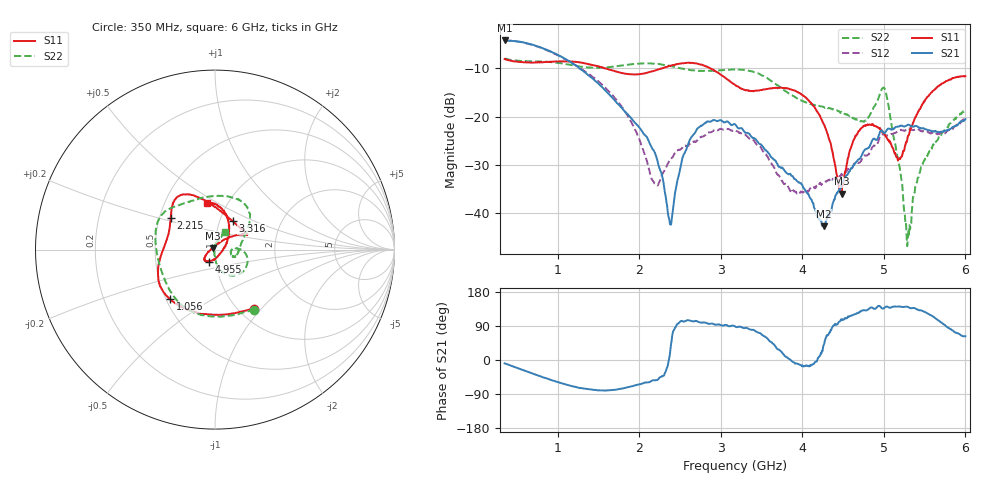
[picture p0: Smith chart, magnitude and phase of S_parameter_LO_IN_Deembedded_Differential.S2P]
!Agilent Technologies,E5071B,MY42403504,A.06.51
!Date: Mon Mar 10 15:44:32 2014
!Data & Calibration Information:
!Freq	S11:SOLT2(ON)	S21:SOLT2(ON)	S12:SOLT2(ON)	S22:SOLT2(ON)
# Hz S dB R 50
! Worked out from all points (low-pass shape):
!   801 points, 350 MHz to 6 GHz, reference 50 ohm
!   highest |S21| = -4.23 dB at 350 MHz (marker M1); lowest = -42.8 dB at 4.263 GHz (marker M2)
!   |S21| within 3 dB of the highest: start of sweep to 1.003 GHz
!   lowest |S11| = -36.0 dB at 4.482 GHz (marker M3), VSWR 1.03, Z = 48.7 + j0.937 ohm
!   |S11| at or under -10 dB: 1.579 GHz to 2.283 GHz (704.5 MHz wide, 36.5 % of centre); 2.871 GHz to end of sweep
!   |S22| runs from -46.8 to -8.0 dB; largest |S21 - S12| = 0.032
!   S11 on the Smith chart (normalised r, x): 350 MHz: 1.17, -0.91; 1.056 GHz: 0.53, -0.34; 2.215 GHz: 0.57, +0.22; 3.316 GHz: 1.15, +0.38; 4.955 GHz: 0.93, -0.13; 6 GHz: 0.81, +0.45
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3.5e8  -8.09 -56.4  -4.23 -8.8  -4.23 -8.4  -7.97 -56.8
1.05625e9  -8.57 -132.0  -7.69 -61.7  -7.82 -60.3  -9.01 -126.1
1.296375e9  -8.85 -150.0  -10.37 -74.3  -10.22 -72.2  -9.67 -146.9
1.826062e9  -11.10 173.2  -18.98 -73.7  -18.98 -83.5  -9.33 166.1
2.2145e9  -10.36 144.4  -28.61 -53.2  -34.12 -6.9  -9.10 144.2
2.235688e9  -10.22 143.1  -30.03 -50.2  -33.98 7.1  -9.10 143.0
2.384e9  -9.46 135.6  -42.37 29.3  -28.77 47.8  -9.55 135.1
2.52525e9  -8.95 129.2  -28.97 103.2  -26.51 63.7  -10.06 126.5
2.645312e9  -8.89 123.1  -24.15 102.3  -25.35 74.4  -10.43 117.5
3.175e9  -13.46 80.0  -21.58 88.5  -22.87 97.0  -10.24 66.5
3.31625e9  -14.52 58.7  -23.38 85.0  -23.96 94.1  -10.43 55.8
3.853e9  -14.34 26.4  -31.84 0.5  -35.47 35.5  -15.44 22.0
4.121375e9  -17.48 35.4  -37.65 -11.8  -34.87 40.0  -17.41 -1.3
4.262625e9  -21.58 45.1  -42.76 39.6  -33.75 53.5  -18.04 -12.5
4.481562e9  -35.98 142.8  -33.96 105.2  -31.85 80.7  -19.04 -21.5
4.679312e9  -23.36 -144.3  -29.05 124.1  -29.61 107.9  -20.63 -16.2
4.95475e9  -22.40 -116.8  -23.10 141.1  -24.11 140.6  -15.23 -7.9
5.060688e9  -24.89 -95.6  -22.47 138.9  -23.78 137.0  -18.08 -74.1
5.194875e9  -28.63 -33.1  -22.01 141.2  -22.86 140.9  -30.56 -97.6
5.300812e9  -23.89 21.9  -21.68 139.5  -22.46 140.2  -43.75 148.5
5.484438e9  -17.19 55.6  -22.39 128.6  -23.01 131.8  -29.44 84.3
6e9  -11.64 99.7  -20.51 62.7  -20.52 66.0  -18.68 59.8
